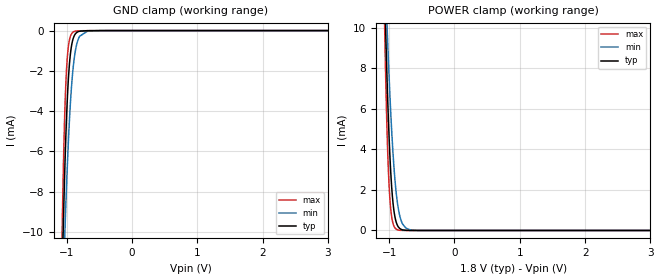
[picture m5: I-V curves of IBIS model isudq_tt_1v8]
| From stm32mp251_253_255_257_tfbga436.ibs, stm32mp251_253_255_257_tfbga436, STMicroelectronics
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[Model]   isudq_tt_1v8
Model_type Input
Polarity   Non-Inverting
Enable   Active-Low
| CAP_THRESHOLD on pad IOTT is "UDTCAPC" :
| Rising=30.0% of vddiov33m   Falling=70.0% of vddiov33m
| C_comp min and max val. don't necessarily correlate with the min and max pvt
| but are the smallest and greatest pad capacitance found.
| var   typ   min   max
C_comp   835.18650fF  767.92500fF  1.02683pF
|C_comp_pullup   436.92000fF  432.03000fF  439.98500fF
|C_comp_pulldown   398.26650fF  335.89500fF  586.84500fF
Vinl = 480.0mV
Vinh = 1.4V
[Model Spec]
| TIME_THRESHOLD on pin ZIV08M is "CMOS" :
| Rising=50.0% of vddv08m   Falling=50.0% of vddv08m
Vinl 1.13970V 1.10770V 1.26170V
Vinh 1.28430V 1.14430V 1.42630V
| variable   typ   min   max
[Temperature Range] 25.0 125.0 -40.0
| variable   typ   min   max
[Voltage Range] 1.8V 1.6V 2.0V
| variable   typ   min   max
[POWER Clamp Reference] 1.8V 1.6V 2.0V
| variable   typ   min   max
[GND Clamp Reference] 0V 0V 0V
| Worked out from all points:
|   GND clamp passes 1 mA (typ) near -0.94 V on its own axis
|   POWER clamp passes 1 mA (typ) near -0.93 V on its own axis
[POWER Clamp]
-1.8V     152.1mA    105.6mA    221.1mA
-1.07V    12.07mA    13.62mA    10.38mA
-1.05V    9.569mA    11.75mA    7.248mA
-1.03V    7.339mA    9.994mA    4.743mA
-1.01V    5.42mA     8.359mA    2.898mA
-990mV    3.841mA    6.86mA     1.662mA
-970mV    2.609mA    5.514mA    906.4uA
-940mV    1.358mA    3.807mA    344uA
-880mV    308.3uA    1.549mA    45.49uA
-790mV    28.48uA    299.8uA    2.102uA
-610mV    226.6nA    8.262uA    7.402nA
3.6V      0A         0A         0A
[GND Clamp]
-1.8V     -182.8mA   -127.8mA   -264.2mA
-1.07V    -12.53mA   -14.65mA   -10.34mA
-1.05V    -9.669mA   -12.45mA   -6.916mA
-1.03V    -7.182mA   -10.39mA   -4.31mA
-1.02V    -6.092mA   -9.426mA   -3.312mA
-1V       -4.24mA    -7.635mA   -1.866mA
-980mV    -2.822mA   -6.045mA   -1mA
-950mV    -1.424mA   -4.065mA   -373.3uA
-890mV    -308.8uA   -1.558mA   -54.59uA
-810mV    -40.51uA   -342.8uA   -10.79uA
-680mV    -5.352uA   -27.64uA   -4.997uA
3.6V      7.948nA    144.9nA    1.008nA
